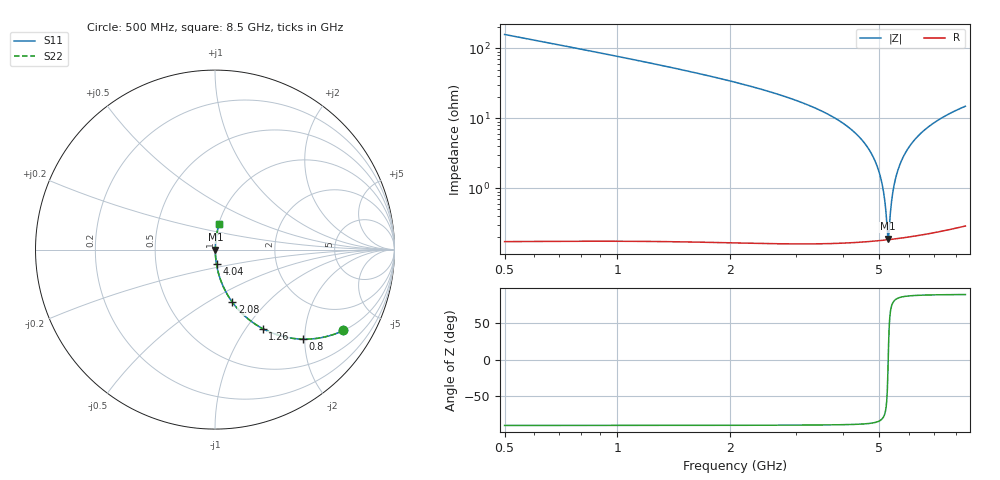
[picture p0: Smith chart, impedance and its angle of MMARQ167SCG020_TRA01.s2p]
! MMARQ167SCG020_TRA01  S-PARAMETER MODEL  ( General Type )
! Model Generated by TAIYO YUDEN Corporation (http://www.ty-top.com)
! Version 1.0
! TAIYO YUDEN Control No. 150305
! Copyright(c) 2015 TAIYO YUDEN CO.,LTD. All Rights Reserved.
! Product Description (link to TY-COMPAS)
! https://ds.yuden.co.jp/TYCOMPAS/or/detail?pn=MMARQ167SCG020BTRA01&u=M
! Products Name : Multilayer Ceramic Capacitors
! Characteristics :
!  Capacitance : 2 pF , Rated Voltage : 250V , TCC : CG / C0G
!  Case Size : 1.6 x 0.8 / 0.063 x 0.031 [mm/inch] , Thickness : 0.7 / 0.028 [mm/inch]
!  (Conditions: Temperature = 25 degC , DC Bias Current/Voltage = 0A / 0V)
! External Node Assignments :
!  1  o---| |---o  2
! GND o---------o GND
! Frequency Range : 500MHz  -  8.5GHz  [ 401 STEP ]
# MHz S RI R 50
! Freq[MHz].  S11 Real  S11 Imag  S21 Real  S21 Imag  S12 Real  S12 Imag  S22 Real  S22 Imag
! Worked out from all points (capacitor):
!   401 points, 500 MHz to 8.5 GHz, reference 50 ohm
!   read as one part in series: C = 1.99 pF near 540 MHz
!   lowest |Z| = 190 mohm at 5.28 GHz (marker M1)
!   series resonance near 5.288 GHz, so ESL is about 460 pH
!   S11 on the Smith chart (normalised r, x): 500 MHz: 1.00, -3.17; 800 MHz: 1.00, -1.96; 1.26 GHz: 1.00, -1.20; 2.08 GHz: 1.00, -0.65; 4.04 GHz: 1.00, -0.17; 8.5 GHz: 1.01, +0.30
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500  0.7155 -0.4506  0.2845 0.4506  0.2845 0.4506  0.7155 -0.4506
800  0.4888 -0.499  0.5112 0.499  0.5112 0.499  0.4888 -0.499
1260  0.265 -0.4399  0.735 0.4399  0.735 0.4399  0.265 -0.4399
1840  0.1288 -0.3328  0.8712 0.3328  0.8712 0.3328  0.1288 -0.3328
2080  0.0971 -0.2935  0.9029 0.2935  0.9029 0.2935  0.0971 -0.2935
3180  0.0267 -0.1564  0.9733 0.1564  0.9733 0.1564  0.0267 -0.1564
4040  0.0084 -0.0818  0.9916 0.0818  0.9916 0.0818  0.0084 -0.0818
4500  0.0041 -0.0489  0.9959 0.0489  0.9959 0.0489  0.0041 -0.0489
4800  0.00261 -0.0293  0.9974 0.0293  0.9974 0.0293  0.00261 -0.0293
5020  0.00204 -0.0157  0.998 0.0157  0.998 0.0157  0.00204 -0.0157
5100  0.00192 -0.011  0.9981 0.011  0.9981 0.011  0.00192 -0.011
5160  0.00187 -0.00743  0.9981 0.00743  0.9981 0.00743  0.00187 -0.00743
5260  0.00184 -0.00162  0.9982 0.00162  0.9982 0.00162  0.00184 -0.00162
5280  0.00184 -0.000478  0.9982 0.000478  0.9982 0.000478  0.00184 -0.000478
5320  0.00185 0.0018  0.9981 -0.0018  0.9981 -0.0018  0.00185 0.0018
5400  0.0019 0.00631  0.9981 -0.00631  0.9981 -0.00631  0.0019 0.00631
5500  0.00203 0.0119  0.998 -0.0119  0.998 -0.0119  0.00203 0.0119
5640  0.0023 0.0195  0.9977 -0.0195  0.9977 -0.0195  0.0023 0.0195
5840  0.00287 0.03  0.9971 -0.03  0.9971 -0.03  0.00287 0.03
6380  0.00536 0.0568  0.9946 -0.0568  0.9946 -0.0568  0.00536 0.0568
7180  0.0111 0.093  0.9889 -0.093  0.9889 -0.093  0.0111 0.093
8500  0.0245 0.1453  0.9755 -0.1453  0.9755 -0.1453  0.0245 0.1453
